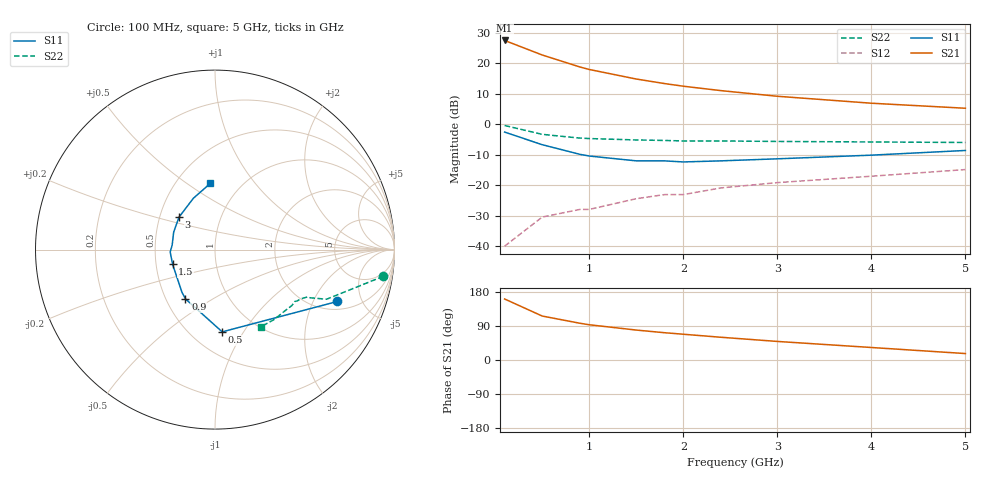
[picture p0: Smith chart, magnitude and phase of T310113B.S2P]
!AT-31011
!S and NOISE PARAMETERS at Vce=2.7V  Ic=10mA.  LAST UPDATED 04-10-94
# ghz s ma r 50
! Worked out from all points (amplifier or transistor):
!   11 points, 100 MHz to 5 GHz, reference 50 ohm
!   highest |S21| = 27.4 dB at 100 MHz (marker M1)
!   |S21| within 3 dB of that: start of sweep to 351.8 MHz
!   unconditionally stable (mu >= 1): 987.8 MHz to 4.914 GHz
!   at 500 MHz: K = 0.65, MSG = 26.6 dB, |S12| = -30.5 dB
!   at 1.8 GHz: K = 1.06, MAG = 16.7 dB, |S12| = -23.1 dB
!   at 5 GHz: K = 0.99, MSG = 10.0 dB, |S12| = -14.9 dB
!   lowest NFmin = 1.30 dB at 500 MHz
!   S11 on the Smith chart (normalised r, x): 100 MHz: 2.44, -3.12; 500 MHz: 0.70, -0.81; 900 MHz: 0.63, -0.38; 1.5 GHz: 0.61, -0.11; 3 GHz: 0.63, +0.25; 5 GHz: 0.73, +0.62
0.1  0.74 -23.0  23.49 161.0  0.01 77.0  0.95 -9.0
0.5  0.46 -85.0  13.57 116.0  0.03 59.0  0.68 -24.0
0.9  0.32 -121.0  8.64 97.0  0.04 59.0  0.59 -27.0
1  0.3 -128.0  7.86 93.0  0.04 59.0  0.58 -27.0
1.5  0.25 -161.0  5.48 79.0  0.06 61.0  0.55 -30.0
1.8  0.25 -177.0  4.62 72.0  0.07 61.0  0.54 -32.0
2  0.24 174.0  4.18 68.0  0.07 61.0  0.53 -33.0
2.4  0.25 157.0  3.54 60.0  0.09 59.0  0.53 -36.0
3  0.27 138.0  2.86 49.0  0.11 58.0  0.52 -40.0
4  0.31 113.0  2.2 33.0  0.14 54.0  0.51 -50.0
5  0.37 94.0  1.82 17.0  0.18 48.0  0.5 -59.0
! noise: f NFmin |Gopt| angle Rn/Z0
0.5  1.3  0.45  11  0.55
0.9  1.4  0.37  33  0.46
1.8  1.7  0.25  86  0.29
2.4  2  0.18  129  0.18
